PROGRAM Communication
VAR
	fbKL6811ConfigNew				:	FB_KL6811ConfigNew;
	fbKL6811Communication			:	FB_KL6811Communication;
	stInData						:	ST_KL6811InData;
	stOutData						:	ST_KL6811OutData;
	bConfigurate					:	BOOL;
END_VAR

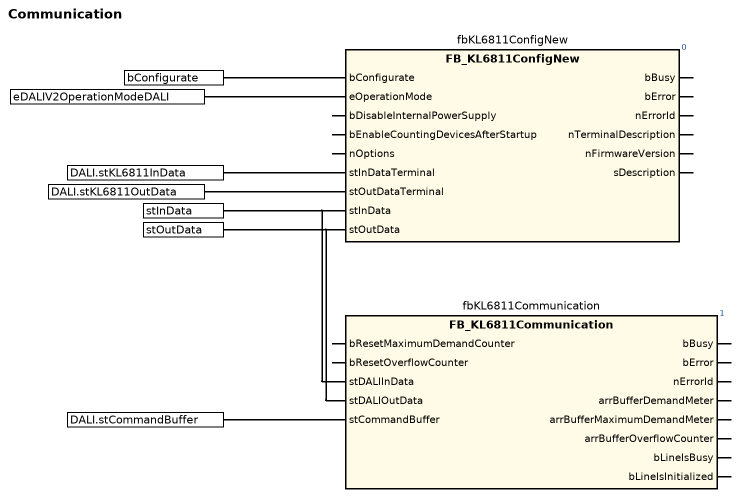
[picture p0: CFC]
fbKL6811ConfigNew(
    bConfigurate := bConfigurate,
    eOperationMode := eDALIV2OperationModeDALI,
    stInDataTerminal := DALI.stKL6811InData,
    stOutDataTerminal := DALI.stKL6811OutData,
    stInData := stInData,
    stOutData := stOutData); // FB_KL6811ConfigNew
fbKL6811Communication(
    stDALIInData := stInData,
    stDALIOutData := stOutData,
    stCommandBuffer := DALI.stCommandBuffer); // FB_KL6811Communication

END_PROGRAM
